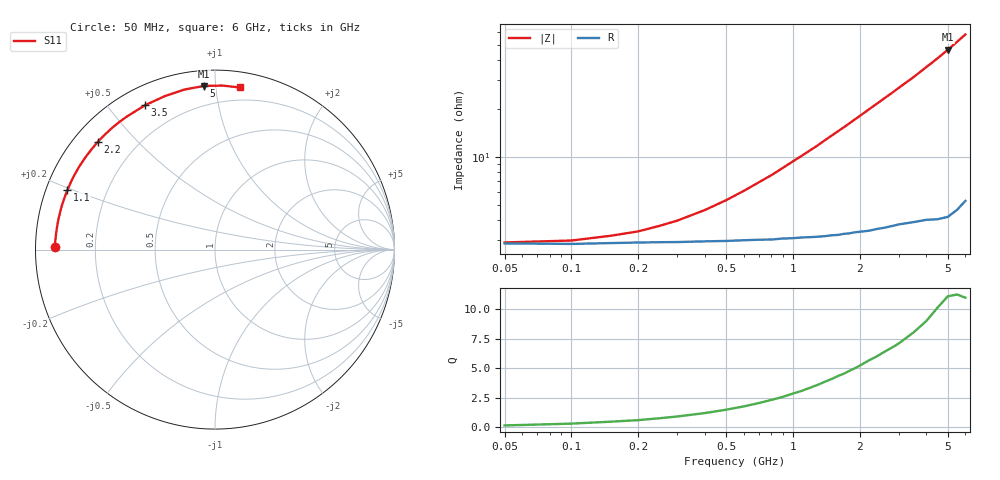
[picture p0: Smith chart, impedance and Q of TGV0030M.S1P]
! SIEMENS Discrete & RF Semiconductors
! BAT64
! Si Schottky Diode in SOT23
! IF = 30 mA
! S-Parameters:  February  1997
# GHz  S  MA  R  50
!  f  S11
! GHz  MAG  ANG
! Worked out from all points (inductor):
!   34 points, 50 MHz to 6 GHz, reference 50 ohm
!   read as one part to ground: L = 1.4 nH near 1.1 GHz
!   highest Q = 11.1 at 5 GHz (marker M1), where L = 1.48 nH
!   S11 on the Smith chart (normalised r, x): 50 MHz: 0.06, +0.01; 1.1 GHz: 0.06, +0.19; 2.2 GHz: 0.07, +0.39; 3.5 GHz: 0.08, +0.62; 5 GHz: 0.08, +0.93; 6 GHz: 0.11, +1.16
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0.05  0.8915 178.9
0.1  0.8923 177.9
0.15  0.8911 176.8
0.2  0.8903 175.9
0.25  0.8899 174.8
0.4  0.889 171.8
0.6  0.888 167.8
0.7  0.8876 165.8
0.8  0.8878 163.9
1  0.8869 159.9
1.1  0.8864 158.0
1.3  0.8867 154.2
1.4  0.8867 152.2
1.6  0.8867 148.4
1.8  0.8864 144.7
1.9  0.886 142.8
2  0.8863 141.0
2.2  0.8872 137.3
2.4  0.8871 133.8
2.6  0.888 130.3
2.8  0.8885 127.0
3  0.8892 123.6
3.5  0.8939 115.8
4  0.8997 108.0
4.5  0.9077 100.9
5  0.9139 93.9
5.5  0.9149 87.4
6  0.9138 81.3
